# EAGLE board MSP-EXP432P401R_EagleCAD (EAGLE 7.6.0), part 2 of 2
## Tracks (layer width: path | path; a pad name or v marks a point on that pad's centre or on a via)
!RST  (via drill 0.3)
  Top 0.203: 54.61,34.29 v54.74,34.42 52.2,34.42 J2.16 | MSP1.83 26.72,23.74 26.29,23.3 25.08,23.3 24.57,22.8 24.57,19.37 24.89,19.05 39.75,19.05 40.96,20.26 45.53,20.26 46.1,19.68 56.2,19.68 57.53,21.02 v57.53,34.42 57.53,43.18 52.58,48.13 52.58,54.1 | J101.11 24.13,51.05 24.64,50.55 37.08,50.55 38.73,52.2 | 38.73,52.2 38.73,52.96 40.48,54.7 C13.1 R6.1 51.98,54.7 52.58,54.1 | 52.58,54.1 54.1,54.1 57.91,57.91 57.91,87.88 56.64,89.15 53.34,89.15 52.07,90.42 49.97,90.42 S3.S1 | J8.10 38.73,52.2
  Bottom 0.203: v57.53,34.42 v54.74,34.42
+3V3  (via drill 0.3)
  Top 0.203: MSP1.13 42.53,32.38 C4.1 42.94,32.77 v44.2,32.77 | v17.53,29.72 17.73,29.51 17.73,28.69 C7.1 17.73,26.73 C3.+ 18.6,27.38 MSP1.73 | R1.1 v19.05,43.31 | R6.2 51.31,53.38 v51.31,52.58
  Top 0.305: 18.91,26.81 C3.+
  Mid-Top 0.508: J5.35 J5.36 49.53,8.41 52.07,10.95 J6.1
  pour Mid-Top (isolate 0.254): 58.42,55.88 15.49,55.88 15.49,52.99 14.7,52.2 12.45,52.2 11.81,51.56 11.81,48.7 11.24,48.13 4.95,48.13 4.32,47.5 4.32,38.94 4.78,38.48 7.67,38.48 8.13,38.02 8.13,28.66 8.85,27.94 18.59,27.94 19.05,28.4 19.05,29.91 19.02,30.48 19.02,40.63 20.3,41.91 29.96,41.91 33.9,45.85 40.42,45.85 41.91,44.36 41.91,32.21 42.37,31.75 50.34,31.75 50.8,31.29 50.8,10.16 51.43,9.53 58.42,9.53
+5V  (via drill 0.3)
  Top 0.508: J5.33 J5.34 46.99,4.32 45.72,5.59 12.19,5.59 J7.1
  other vias: 8.13,49.91 9.4,49.91
  pour Mid-Top (isolate 0.61, rank 2): 0,55.88 14.99,55.88 14.99,53.57 14.37,52.96 11.79,52.96 11.05,52.22 11.05,49.81 10.51,49.28 4.3,49.28 3.56,48.54 3.56,38.35 4.19,37.72 6.83,37.72 7.37,37.19 7.62,9.99 7.16,9.53 0,9.53
  pour Bottom (isolate 0.254): 7.24,43.05 10.74,43.05 11.3,43.62 11.3,50.11 10.74,50.67 7.52,50.67 7.24,50.39
AVCC
  Top 0.203: MSP101.6 39.43,80.03 39.02,79.63 36.14,79.63 35.81,79.3 35.81,78.74 C116.2 35.77,78.71 35.72,78.71 R115.1 R114.2
AVCCOUT  (via drill 0.3)
  Top 0.203: R113.1 43.95,78.11 43.94,78.11 43.94,77.09 43.96,77.09 R112.2 | R113.1 44.16,78.99 v44.88,78.99 | 43.92,82.09 43.92,82.07 43.97,82.02 43.99,82.04 | 43.99,81.95 43.99,82.04 | 43.99,82.04 43.99,82.07 43.97,82.09 | C115.2 43.92,82.13 43.2,81.41 43.2,79.67 R113.1 | 43.81,78.97 43.9,78.97 R113.1 | MSP101.1 35.6,83.27 v35.56,83.57
  Top 0.508: C115.2 43.94,82.12 43.92,82.09
  Bottom 0.203: v35.56,83.57 35.56,82.3 37.34,80.52 43.36,80.52 v44.88,78.99
DCDCCAL0
  Top 0.203: R126.2 45.83,80.52 45.47,80.9 45.11,81.26 45.11,84.71 44.35,85.47 43.23,85.47 42.42,84.66 42.42,83.66 42.03,83.27 MSP101.12
DCDCCAL1  (via drill 0.3)
  Top 0.203: R127.2 45.8,77.64 45.8,78 45.8,78.46 45.82,78.49 45.8,78.49 v45.8,78.54 | MSP101.2 37.39,82.62 37.21,82.8 36.07,82.8 35.94,82.68 35.05,82.68 v34.92,82.55
  Bottom 0.203: v45.8,78.54 45.64,78.54 45.21,78.11 44.2,78.11 43.69,78.61 43.69,78.74 42.42,80.01 37.21,80.01 34.92,82.3 v34.92,82.55
DCDCCAL2
  Top 0.203: 41.62,82.63 MSP101.11 42.42,82.62 42.93,83.13 42.93,84.42 43.46,84.96 44.06,84.96 44.68,84.35 44.68,80.33 45.55,79.45 R128.2
DCDCIO0  (via drill 0.3)
  Top 0.203: MSP101.4 35.69,81.32 34.29,79.92 34.29,68.15 33.7,67.56 v30.73,67.56 | v21.46,68.2 20.83,68.83 12.66,68.83 11.81,67.98 IC106.P$5
  Bottom 0.203: v30.73,67.56 22.1,67.56 v21.46,68.2
DCDCIO1  (via drill 0.3)
  Top 0.203: MSP101.5 38.78,80.14 38.64,80.01 35.26,80.01 34.8,79.55 34.8,67.62 34.23,67.06 31.53,67.06 31.11,66.65 v30.86,66.55 | v20.07,68.2 12.83,68.2 12.21,67.58 IC106.P$6
  Bottom 0.203: v30.86,66.55 21.72,66.55 v20.07,68.2
DCDCPULSE  (via drill 0.3)
  Top 0.203: R118.2 45.82,84.95 v45.82,84.66 | MSP101.3 36.9,81.97 v36.83,82.04 35.59,82.04 33.78,80.24 33.78,69.25 32.86,68.33 30.35,68.33 v30.1,68.58 | v21.08,70.23 12.7,70.23 10.18,67.71 IC106.P$127
  Bottom 0.203: v36.83,82.04 37.72,81.15 42.32,81.15 v45.82,84.66 | v21.08,70.23 21.34,70.23 22.99,68.58 v30.1,68.58
DCDCRST  (via drill 0.3)
  Top 0.203: MSP101.9 41.91,81.32 42.19,81.04 42.19,78.64 TP108.1 42.16,77.85 38.48,74.17 36.2,74.17 v35.56,73.53 | IC106.P$11 14.21,64.91 14.73,64.39 18.41,64.39 v18.54,64.26
  Bottom 0.203: v18.54,64.26 18.8,64.26 19.94,65.41 35.56,65.41 36.07,65.91 36.07,67.56 35.56,68.07 v35.56,73.53
DCDCTEST  (via drill 0.3)
  Top 0.203: 41.73,81.97 41.66,82.04 41.66,81.92 MSP101.10 42.18,81.97 42.7,81.45 42.7,79.6 43.31,78.99 43.31,77.85 42.16,76.71 TP109.1 | TP109.1 | IC106.P$27 20.61,64.68 v20.07,64.14 | TP109.1 41.27,76.07 38.48,73.28 v36.7,73.28
  Bottom 0.203: v20.07,64.14 20.96,65.02 36.32,65.02 36.7,65.41 v36.7,73.28
DCOR
  Top 0.203: MSP1.44 26.21,41.1 24.13,43.18 R5.1
HOSTSCL  (via drill 0.3)
  Top 0.203: R117.2 39.15,78.65 39.88,79.38 v40,79.38 40.08,79.45 MSP101.7 | IC106.P$49 25,73.71 25.4,73.31 25.4,70.99 25.91,70.48 32.64,70.48 33.02,70.87 33.02,72.64 v32.77,72.9
  Bottom 0.203: v40,79.38 39.88,79.25 36.83,79.25 35.05,77.47 35.05,75.69 33.78,74.42 33.78,73.66 33.02,72.9 v32.77,72.9
HOSTSDA  (via drill 0.3)
  Top 0.203: 40.2,78.26 R116.2 40.28,78.26 v40.77,78.74 40.73,78.74 MSP101.8 | IC106.P$50 25.19,74.11 25.78,73.52 25.78,71.63 26.29,71.12 31.75,71.12 v32,71.37
  Bottom 0.203: v40.77,78.74 40.51,78.49 36.83,78.49 35.81,77.47 35.81,75.44 34.54,74.17 34.54,73.66 32.26,71.37 v32,71.37
IRSTN  (via drill 0.3)
  Top 0.203: R102.1 32.26,73.53 v30.48,71.76 | v4.7,72.77 3.43,72.77 TP106.1
  Bottom 0.203: v4.7,72.77 7.37,72.77 8.26,73.66 21.34,73.66 24.26,70.74 29.46,70.74 v30.48,71.76
ITCK
  Top 0.203: IC106.P$100 4.17,78.51 3.61,79.07 R129.1 2.84,79.72 2.54,80.01 2.54,80.77 1.27,82.04 TP103.1
ITDI  (via drill 0.3)
  Top 0.203: IC106.P$98 5.65,79.31 v5.33,79.63
  Bottom 0.203: v5.33,79.63 3.43,79.63 TP105.1
ITDO  (via drill 0.3)
  Top 0.203: IC106.P$97 6.27,79.71 v5.33,80.65
  Bottom 0.203: v5.33,80.65 1.9,80.65 TP104.1
ITMS
  Top 0.203: IC106.P$99 4.9,78.91 4.57,79.24 4.57,83.12 3.85,83.84 R125.1 2.38,85.09 TP102.1
LED0  (via drill 0.3)
  Top 0.203: IC106.P$3 11.01,64.61 v9.65,63.25 | R111.1 4.66,63.92 v4.83,63.75
  Bottom 0.203: v9.65,63.25 5.33,63.25 v4.83,63.75
LED1  (via drill 0.3)
  Top 0.203: IC106.P$4 11.41,64.5 10.54,63.63 v10.54,62.61 | v4.06,62.74 3.97,62.83 R124.1
  Bottom 0.203: v10.54,62.61 10.41,62.48 4.32,62.48 v4.06,62.74
N$1
  Top 0.254: JP102.2 48.39,59.56 J102.1
N$3
  Top 0.203: IC106.P$63 25.84,79.31 28.7,76.45 R108.2
N$4
  Top 0.203: R124.2 1.71,62.56 3.56,60.71 3.56,58.87 LED102.A
N$6  (via drill 0.3)
  Top 0.203: 32,22.29 C2.1 | 21.16,43.27 R1.2
  Top 0.305: 32,22.29 32,22.86 31.5,23.37 29.08,23.37 28.7,23.75 MSP1.87 28.7,26.12 28.47,26.35 v27.81,26.35 | 21.16,43.27 C1.1 22.73,42.67 23.37,42.04 24.64,42.04 25.71,40.97 MSP1.45 25.71,38.26 26.12,37.85 27.62,37.85 v27.81,38.04
  Bottom 0.305: v27.81,26.35 v27.81,38.04
N$7
  Top 0.203: LED101.A 2.72,60.53 2.29,60.96 1.27,60.96 0.76,61.47 0.76,63.5 1.18,63.92 R111.2
N$8
  Top 0.203: JP9.2 28.36,10.58 R2.1
N$9
  Top 0.203: R2.2 30.7,7.49 35.43,7.49 35.94,8 35.94,8.76 36.2,9.02 LED2.5
N$10
  Top 0.203: R3.2 32.86,7.87 35.18,7.87 35.56,8.26 35.56,9.27 36.03,9.74 LED2.6
N$11  (via drill 0.3)
  Top 0.203: R4.2 34.92,8.93 v34.92,9.65 | v36.58,7.49 36.66,7.58 LED2.4
  Bottom 0.203: v34.92,9.65 36.58,8 v36.58,7.49
N$12
  Top 0.305: R119.1 47.15,81.78 47.5,81.43 48.62,81.43 48.67,81.38 T102.E
N$13
  Top 0.305: T102.B 48.72,83.72 D101.2 D101.1 48.05,87.29 46.92,86.17 R118.1 46.8,85.74
N$15  (via drill 0.3)
  Top 0.635: D102.3 50.8,78.79 v51.61,79.38 | T101.3 55.37,81.05 v55.37,79.88 55.37,78.77 L101.1
  Bottom 0.635: v51.61,79.38 54.86,79.38 v55.37,79.88
N$16
  Top 0.203: 50.92,82.38 T102.C
  Top 0.305: T102.C 52.67,82.37 T101.1 | 50.98,82.32 50.92,82.38 D101.3 50.95,86.31 52.35,86.31 52.73,85.93 R120.2
N$17
  Top 0.203: LED1.A R7.2
N$19
  Top 0.203: JP10.2 30.9,10.58 R3.1
N$21
  Top 0.203: IC106.P$93 11.41,82.39 9.91,83.89 R138.2
N$22
  Top 0.203: IC106.P$61 24.99,78.51 26.92,76.58 R110.2
N$23
  Top 0.203: IC106.P$95 10.61,82.01 9.06,83.57 8.64,83.57 8.13,84.07 R131.2
N$24
  cutout Mid-Bottom: 11.68,86.28 17.53,86.36 17.53,82.27 11.66,82.25
  cutout Top: 11.68,86.28 17.53,86.36 17.53,82.27 11.66,82.25
  cutout Bottom: 11.68,86.28 17.53,86.36 17.53,82.27 11.66,82.25
  cutout Mid-Top: 11.68,86.28 17.53,86.36 17.53,82.27 11.66,82.25
N$25
  Top 0.203: JP11.2 33.44,10.58 R4.1
N$27
  Top 0.203: IC106.P$62 25.36,78.91 27.81,76.45 R109.2
N$29
  Top 0.254: JP8.2 24.13,9.17 R7.1
N$30
  cutout Top: 31.24,22.99 25.4,22.99 25.02,22.61 25.02,19.81 25.27,19.56 31.11,19.56 31.37,19.81 31.37,22.86
N$31
  cutout Mid-Top: 25.4,22.99 25.02,22.61 25.02,19.81 25.27,19.56 31.11,19.56 31.37,19.81 31.37,22.86 31.24,22.99
N$32
  cutout Mid-Bottom: 25.4,22.99 25.02,22.61 25.02,19.81 25.27,19.56 31.11,19.56 31.37,19.81 31.37,22.86 31.24,22.99
N$33
  cutout Bottom: 25.4,22.99 25.02,22.61 25.02,19.81 25.27,19.56 31.11,19.56 31.37,19.81 31.37,22.86 31.24,22.99
N$34
  Top 0.203: MSP1.42 27.2,41.38 26.49,42.09 Q1.1 26.47,43.46 C6.1
N$35
  cutout Mid-Top: 25.02,46.61 25.02,42.93 26.67,41.27 26.67,39.37 27.05,38.99 28.07,38.99 28.32,39.24 28.32,41.15 29.72,42.54 29.72,46.61 28.83,47.5 25.91,47.5
N$36
  cutout Mid-Bottom: 25.91,47.5 25.02,46.61 25.02,42.93 26.67,41.27 26.67,39.37 27.05,38.99 28.07,38.99 28.32,39.24 28.32,41.15 29.72,42.54 29.72,46.61 28.83,47.5
N$37
  cutout Bottom: 25.91,47.5 25.02,46.61 25.02,42.93 26.67,41.27 26.67,39.37 27.05,38.99 28.07,38.99 28.32,39.24 28.32,41.15 29.72,42.54 29.72,46.61 28.83,47.5
N$38
  Top 0.203: MSP1.41 27.71,41.43 28.4,42.11 Q1.2 28.35,43.48 C5.1
N$47
  Top 0.203: IC106.P$59 25.16,77.71 26.04,76.84 R139.2
OSC0
  Top 0.203: C102.1 16.58,85.6 Q101.3 15.24,85.6 14.61,84.96 14.61,83.19 13.41,81.99 IC106.P$88
OSC1
  Top 0.203: IC106.P$89 13.01,81.98 12.33,82.67 R106.2
OSC1_R
  Top 0.203: R106.1 13.51,83.17 Q101.1 12.58,84 C101.1
P1.0_LED1  (via drill 0.3)
  Top 0.203: v38.04,14.86 37.65,14.48 36.64,14.48 36.13,14.99 26.48,14.99 25.46,13.97 JP8.1 | MSP1.4 38.3,27.89 v38.35,27.94
  Bottom 0.203: v38.04,14.86 38.73,15.56 38.73,20.57 39.12,20.96 39.12,27.3 38.48,27.94 v38.35,27.94
P1.1_BUTTON1  (via drill 0.3)
  Top 0.203: MSP1.5 35.51,28.4 v35.05,27.94 | v17.53,42.67 17.53,45.21 9.91,52.83 S1.S1
  Mid-Top 0.203: v17.53,42.67 18.54,41.66 18.54,40.64 21.08,38.1 23.37,38.1 29.46,32 30.99,32 v35.05,27.94
P1.2_BCLUART_RXD  (via drill 0.3)
  Top 0.203: MSP1.6 35.21,28.88 34.42,29.68 34.42,36.07 34.92,36.58 v34.92,37.59 | v32.51,47.24 31.75,48.01 30.73,48.01 29.72,49.02 20.32,49.02 19.05,50.29 J101.7
  Mid-Top 0.203: v34.92,37.59 32.51,40 v32.51,47.24
P1.3_BCLUART_TXD  (via drill 0.3)
  Top 0.203: MSP1.7 35.76,29.39 34.8,30.35 34.8,35.5 v35.24,35.94 | v33.27,48.39 33.15,48.51 31.24,48.51 29.97,49.78 22.61,49.78 21.59,50.8 J101.9
  Mid-Top 0.203: v35.24,35.94 35.69,36.39 35.69,37.97 33.27,40.39 v33.27,48.39
P1.4_BUTTON2  (via drill 0.3)
  Top 0.203: MSP1.8 37.92,29.9 v38.61,29.21 | v42.67,43.18 46.48,46.99 v49.78,46.99 | S2.S1 55.12,48.2 v55.12,46.74
  Mid-Top 0.203: v38.61,29.21 38.61,30.99 42.16,34.54 42.16,42.67 v42.67,43.18
  Bottom 0.203: v49.78,46.99 50.04,46.74 v55.12,46.74
P1.5_SPICLK_J1.7  (via drill 0.3)
  Top 0.203: v40.13,12.51 38.42,12.51 38.04,12.89 20.7,12.89 20.19,12.38 11.43,12.38 9.08,14.73 9.08,18.61 8.38,19.3 5.02,19.3 4.38,19.94 4.38,28.26 5.33,29.21 J1.7 | MSP1.9 39.22,30.38 39.5,30.1 39.5,27.69 v40.89,26.29
  Bottom 0.203: v40.13,12.51 40.7,13.08 40.7,14.73 40.89,14.92 v40.89,26.29
P1.6_SPIMOSI_J2.15  (via drill 0.3)
  Top 0.203: v48.01,30.29 48.2,30.48 50.8,30.48 J2.15 | MSP1.10 39.22,30.89 39.88,30.23 39.88,27.81 40.64,27.05 47.43,27.05 v47.75,26.73
  Bottom 0.203: v47.75,26.73 48.01,26.99 v48.01,30.29
P1.7_SPIMISO_J2.14
  Top 0.203: MSP1.11 39.22,31.39 40.26,30.35 40.26,27.94 40.64,27.56 44.45,27.56 44.83,27.94 50.8,27.94 J2.14
P2.0_RGBLED_RED  (via drill 0.3)
  Top 0.203: v29.84,32.96 29.84,30.54 26.23,26.92 24.07,26.92 20.7,23.56 20.7,22.1 21.4,21.4 v21.59,21.4 | MSP1.16 37.68,33.88 37.99,33.58 v39.05,33.58
  Bottom 0.203: v39.05,33.58 38.48,32.96 v29.84,32.96 | v21.59,21.4 21.78,21.21 21.78,16.13 22.67,15.24 27.88,15.24 29.15,13.97 JP9.1
P2.1_RGBLED_GREEN  (via drill 0.3)
  Top 0.203: MSP1.17 38.19,34.39 v38.35,34.23 | v29.96,33.92 29.65,33.92 29.08,33.4 29.08,30.35 26.04,27.3 23.88,27.3 19.94,23.37 19.94,22.1 20.64,21.4 v20.64,21.15
  Bottom 0.203: v38.35,34.23 36.77,34.23 35.94,33.4 30.48,33.4 v29.96,33.92 | v20.64,21.15 21.27,20.51 21.27,14.92 23.3,12.89 30.29,12.89 31.37,13.97 JP10.1
P2.2_RGBLED_BLUE  (via drill 0.3)
  Top 0.203: v39.37,34.73 39.26,34.87 39.14,34.99 37.85,34.99 37.72,34.86 37.34,34.86 37.32,34.87 MSP1.18 | v29.84,35.05 28.45,33.65 28.45,30.42 26.61,28.57 v23.81,28.57 | v20.7,25.46 20.45,25.46 19.56,24.57 v19.56,20.96
  Bottom 0.203: v29.84,35.05 30.16,35.05 31.37,33.84 35.69,33.84 36.83,34.99 39.18,34.99 v39.37,34.73 | v19.56,20.96 20.83,19.68 20.83,14.48 22.8,12.51 33.15,12.51 34.29,13.65 JP11.1 | v23.81,28.57 v20.7,25.46
P2.3_IO_J4.34
  Top 0.203: MSP1.19 39.8,35.38 40.51,34.67 42.25,34.67 43.08,33.84 44.64,33.84 45.02,33.46 45.02,30.54 46.35,29.21 J4.34
P2.4_PWM_J4.38
  Top 0.203: MSP1.20 39.19,35.89 42.67,39.37 J4.38
P2.5_PWM_J2.19
  Top 0.203: MSP1.21 39.04,36.37 43.31,40.64 50.8,40.64 J2.19
P2.6_PWM_J4.39
  Top 0.203: MSP1.22 38.91,36.88 43.94,41.91 J4.39
P2.7_PWM_J4.40
  Top 0.203: MSP1.23 38.72,37.39 45.78,44.45 J4.40
P3.0_IO_J2.18  (via drill 0.3)
  Top 0.203: MSP1.32 32.21,41.86 34.29,43.94 37.59,43.94 40.51,41.02 v41.02,41.02
  Bottom 0.203: v41.02,41.02 44.58,41.02 47.5,38.1 50.8,38.1 J2.18
P3.2_URXD_J1.3  (via drill 0.3)
  Top 0.203: MSP1.34 31.22,38.01 29.65,36.45 v26.92,36.45 | v13.46,38.54 11.37,40.64 7.62,40.64 J1.3 | v21.46,39.12 17.34,39.12 v17.08,38.86
  Bottom 0.203: v17.08,38.86 13.78,38.86 v13.46,38.54 | v26.92,36.45 24.13,36.45 v21.46,39.12
P3.3_UTXD_J1.4  (via drill 0.3)
  Top 0.203: MSP1.35 30.71,38.2 29.59,37.08 v26.16,37.08 | v16.19,38.23 16.19,39.24 17.08,40.13 v22.1,40.13 | v11.56,37.85 11.3,38.1 7.62,38.1 J1.4
  Bottom 0.203: v11.56,37.85 15.81,37.85 v16.19,38.23 | v26.16,37.08 25.15,37.08 v22.1,40.13
P3.5_IO_J4.32
  Top 0.203: MSP1.37 29.72,40.96 36.77,48.01 50.6,48.01 55.63,42.98 55.63,23.37 55.12,22.86 50.8,22.86 J4.32
P3.6_IO_J2.11
  Top 0.203: MSP1.38 29.21,40.96 36.7,48.45 50.87,48.45 56.2,43.12 56.2,22.16 55.63,21.59 J2.11
P3.7_IO_J4.31
  Top 0.203: MSP1.39 28.77,41.02 36.7,48.96 51.04,48.96 56.77,43.23 56.77,21.34 55.75,20.32 50.8,20.32 J4.31
P4.0_A13_J3.24
  Top 0.203: MSP1.56 11.67,35.89 10.73,36.83 J3.24
P4.1_IO_J1.5
  Top 0.203: MSP1.57 10.91,35.38 10.73,35.56 7.62,35.56 J1.5
P4.2_A11_J3.25
  Top 0.203: MSP1.58 9.47,34.87 J3.25
P4.3_A10_J1.6
  Top 0.203: MSP1.59 12.68,34.39 11.3,33.02 7.62,33.02 J1.6
P4.4_A9_J3.26
  Top 0.203: MSP1.60 13.12,33.88 10.92,31.69 8.95,31.69 J3.26
P4.5_A8_J3.27
  Top 0.203: MSP1.61 14.9,33.38 10.73,29.21 J3.27
P4.6_IO_J1.8
  Top 0.203: MSP1.62 15.37,32.89 10.41,27.94 7.62,27.94 J1.8
P4.7_A6_J3.28
  Top 0.203: MSP1.63 15.81,32.38 10.1,26.67 J3.28
P5.0_IO_J2.13  (via drill 0.3)
  Top 0.203: MSP1.64 24.89,31.88 26.92,29.84 v26.92,29.78 | v24.77,17.14 46.35,17.14 46.99,17.78 v46.99,18.35 | v47.05,25.34 50.74,25.34 J2.13
  Bottom 0.203: v46.99,18.35 46.99,25.15 v47.05,25.34 | v24.77,17.14 23.62,17.14 23.11,17.65 23.11,22.48 24,23.37 24,26.35 24.77,27.11 25.02,27.11 26.92,29.02 v26.92,29.78
P5.1_IO_J4.33  (via drill 0.3)
  Top 0.203: v23.88,16.51 46.48,16.51 47.62,17.65 v47.62,19.05 | MSP1.65 24.49,31.39 26.04,29.84 v26.04,29.21
  Bottom 0.203: v47.62,19.05 47.62,24.77 J4.33 | v23.88,16.51 23.5,16.51 22.73,17.27 22.73,22.61 23.62,23.5 23.62,26.54 26.04,28.96 v26.04,29.21
P5.2/XT2IN
  Top 0.203: MSP1.86 28.22,23.47 29.29,22.39 Q2.1 | 29.21,22.35 Q2.1 | C12.1 29.48,22.32 Q2.1
P5.2_IO_J2.12  (via drill 0.3)
  Top 0.203: MSP1.66 23.85,30.89 v25.08,29.65 | v25.08,15.88 46.48,15.88 48.32,17.72 v48.32,18.29
  Bottom 0.203: v48.32,18.29 48.32,22.36 48.82,22.86 50.8,22.86 J2.12 | v25.08,15.88 23.37,15.88 22.29,16.95 22.29,22.8 23.24,23.75 23.24,26.8 25.08,28.64 v25.08,29.65
P5.3  (via drill 0.3)
  Top 0.203: MSP1.67 20.68,30.38 v19.68,31.37
  Bottom 0.203: v19.68,31.37 14.86,31.37 14.1,30.61 14.1,18.54 11.05,15.49 11.05,8.89 15.24,4.7 15.24,2.54 J5.9
P5.3/XT2OUT
  Top 0.203: MSP1.85 27.71,23.34 28.19,22.86 28.19,21.33 27.4,20.54 Q2.3 26.91,20.36 C11.1
P5.4_IO_J3.29
  Top 0.203: MSP1.68 20.08,29.9 18.73,31.24 16,31.24 12.38,27.62 12.38,25.08 11.43,24.13 J3.29
P5.5_IO_J3.30
  Top 0.203: MSP1.69 19.89,29.39 18.54,30.73 16.45,30.73 13.27,27.56 13.27,22.92 11.94,21.59 J3.30
P5.6_PWM_J4.37  (via drill 0.3)
  Top 0.203: v40.32,36.07 41.08,36.83 J4.37 | MSP1.70 22.53,28.88 22.86,29.21 22.86,29.91 v23.18,30.23 | v25.72,32.77 25.97,32.77 29.21,36.07 30.58,36.07 v31.22,35.43
  Bottom 0.203: v40.32,36.07 36.39,36.07 35.5,35.18 32.77,35.18 32.51,35.43 v31.22,35.43 | v25.72,32.77 v23.18,30.23
P5.7_IO_J2.17  (via drill 0.3)
  Top 0.203: v41.02,35.37 41.27,35.56 50.8,35.56 J2.17 | v32.13,34.61 30.8,34.61 30.54,34.86 30.54,35.43 30.29,35.69 29.53,35.69 25.96,32.12 v25.96,31.8 | MSP1.71 22.68,28.4 23.81,29.53 v24,29.53
  Bottom 0.203: v32.13,34.61 35.62,34.61 36.39,35.37 v41.02,35.37 | 25.96,31.67 v25.96,31.8 25.96,31.48 v24,29.53
P6.0_A15_J1.2
  Top 0.203: MSP1.54 16.65,36.88 10.35,43.18 7.56,43.18 6.35,41.97 J1.2
P6.1_A14_J3.23
  Top 0.203: MSP1.55 14.24,36.37 11.24,39.37 J3.23
P6.2  (via drill 0.3)
  Top 0.203: MSP1.76 23.22,24.61 v21.97,23.37
  Bottom 0.203: v21.97,23.37 16.38,23.37 15.49,22.48 15.49,18.03 12.45,14.99 12.45,9.65 16.26,5.84 17.27,5.84 19.05,4.06 J5.12
P6.3  (via drill 0.3)
  Top 0.203: MSP1.77 23.7,23.82 22.35,22.48 v21.34,22.48
  Bottom 0.203: v21.34,22.48 16.51,22.48 16,21.97 16,17.78 12.83,14.61 12.83,9.91 16.38,6.35 18.41,6.35 20.32,4.45 20.32,2.41 21.46,1.27 J5.13
P6.4_I2CSDA_J1.10
  Top 0.203: MSP1.78 24.21,23.64 23.75,23.18 23.75,21.34 22.73,20.32 7.62,20.32 J1.10
P6.5_I2CSCL_J1.9
  Top 0.203: MSP1.79 24.71,23.44 24.13,22.86 24.13,21.08 22.86,19.81 5.84,19.81 5.08,20.57 5.08,22.86 J1.9
P6.6_CAPTURE_J4.36  (via drill 0.3)
  Top 0.203: v23.94,17.78 45.47,17.78 46.16,18.48 v46.16,18.99 | v47.05,32.51 47.05,33.84 47.5,34.29 J4.36 | MSP1.80 25.22,25.58 v24.83,26.16
  Bottom 0.203: v24.83,26.16 24.83,23.62 23.5,22.29 23.5,18.22 v23.94,17.78 | v47.05,32.51 47.24,32.32 47.24,27.18 46.42,26.35 46.42,19.24 v46.16,18.99
P6.7_CAPTURE_J4.35  (via drill 0.3)
  Top 0.203: MSP1.81 25.71,26.21 v25.78,26.29 | v46.55,30.99 47.31,31.75 J4.35 | v45.27,19.43 44.26,18.41 v24.64,18.41
  Bottom 0.203: v25.78,26.29 25.78,24.07 24.07,22.35 24.07,18.99 v24.64,18.41 | v46.55,30.99 46.74,30.8 46.74,27.3 45.78,26.35 45.78,19.88 45.34,19.43 v45.27,19.43
P7.0  (via drill 0.3)
  Top 0.203: MSP1.88 29.21,26.54 v28.7,27.05
  Mid-Top 0.203: v28.7,27.05 24.77,27.05 17.65,19.94 17.65,8.64 19.94,6.35 23.37,6.35 25.4,4.32 25.4,2.67 26.67,1.4 J5.17
P7.1  (via drill 0.3)
  Top 0.203: MSP1.89 29.72,27.18 v28.7,28.19
  Mid-Top 0.203: v28.7,28.19 28.45,28.19 27.69,27.43 24.64,27.43 17.27,20.07 17.27,8.38 19.68,5.97 22.1,5.97 24.13,3.94 J5.16
P7.2  (via drill 0.3)
  Top 0.203: MSP1.90 30.2,27.58 v29.84,27.94
  Mid-Top 0.203: v29.84,27.94 29.84,28.32 29.34,28.83 28.32,28.83 27.3,27.81 24.51,27.81 16.89,20.19 16.89,8.13 19.43,5.59 21.46,5.59 22.86,4.19 22.86,2.41 24,1.27 J5.15
P7.3  (via drill 0.3)
  Top 0.203: MSP1.91 30.71,28.47 v29.84,29.34
  Mid-Top 0.203: v29.84,29.34 28.32,29.34 27.18,28.19 24.38,28.19 16.51,20.32 16.51,7.87 19.3,5.08 20.45,5.08 21.59,3.94 J5.14
P7.4  (via drill 0.3)
  Top 0.203: MSP1.26 35.71,40.51 v36.07,40.51
  Mid-Top 0.203: J5.24 34.29,4.57 36.58,6.86 40.26,6.86 41.66,8.26 41.66,19.81 36.2,25.27 36.2,35.31 36.96,36.07 36.96,39.62 v36.07,40.51
P7.5  (via drill 0.3)
  Top 0.203: MSP1.27 34.72,40.95 35.05,41.27 v36.96,41.27
  Mid-Top 0.203: J5.23 35.56,2.54 35.56,4.57 37.46,6.48 40.51,6.48 42.04,8 42.04,20.07 36.58,25.53 36.58,35.18 37.34,35.94 37.34,40.77 36.96,41.15 v36.96,41.27
P7.6  (via drill 0.3)
  Top 0.203: MSP1.28 34.21,41.58 34.54,41.91 v36.07,41.91
  Mid-Top 0.203: J5.26 36.83,4.57 38.35,6.1 40.77,6.1 42.42,7.75 42.42,20.32 36.96,25.78 36.96,35.05 37.72,35.81 37.72,39.88 38.23,40.39 38.23,41.53 37.85,41.91 v36.07,41.91
P7.7  (via drill 0.3)
  Top 0.203: MSP1.29 33.71,42.09 34.16,42.54 36.83,42.54 v36.96,42.67
  Mid-Top 0.203: J5.25 38.1,2.54 38.1,4.57 39.24,5.71 41.02,5.71 42.8,7.49 42.8,20.57 37.34,26.04 37.34,34.92 38.1,35.69 38.1,39.75 38.61,40.26 38.61,42.16 38.1,42.67 v36.96,42.67
P8.0  (via drill 0.3)
  Top 0.203: MSP1.30 33.2,42.34 34.29,43.43 35.81,43.43 v36.07,43.18
  Mid-Top 0.203: v36.07,43.18 36.45,43.56 38.23,43.56 38.99,42.8 38.99,40 38.48,39.5 38.48,35.43 37.72,34.67 37.72,26.29 43.18,20.83 43.18,12.83 v43.69,12.32
  Bottom 0.203: v43.69,12.32 43.69,12.07 40,8.38 39.5,8.38 36.32,5.21 33.27,5.21 31.88,3.81 J5.22
P8.2  (via drill 0.3)
  Top 0.203: MSP1.46 25.22,35.64 v24.89,35.31
  Bottom 0.203: v24.89,35.31 24.89,35.05 24.13,34.29 14.35,34.29 13.59,33.53 13.59,18.8 10.54,15.75 10.54,7.37 13.97,3.94 J5.8
P8.3  (via drill 0.3)
  Top 0.203: MSP1.47 24.71,36.27 v23.5,35.05
  Bottom 0.203: v23.5,35.05 13.46,35.05 13.08,34.67 13.08,19.05 10.03,16 10.03,6.99 12.7,4.32 12.7,2.41 13.84,1.27 J5.7
P8.4  (via drill 0.3)
  Top 0.203: MSP1.48 24.21,36.91 v23.37,36.07
  Bottom 0.203: v23.37,36.07 13.34,36.07 12.57,35.31 12.57,19.3 9.53,16.26 9.53,6.22 11.43,4.32 J5.6
P8.5  (via drill 0.3)
  Top 0.203: MSP1.49 23.7,40.95 22.99,41.66 13.84,41.66 v13.72,41.53
  Bottom 0.203: v13.72,41.53 11.43,41.53 10.16,40.26 10.16,20.19 7.62,17.65 7.62,10.54 6.22,9.14 6.22,3.94 J5.2
P8.6  (via drill 0.3)
  Top 0.203: MSP1.50 23.22,40.66 22.73,41.15 14.86,41.15 v14.22,40.51
  Bottom 0.203: v14.22,40.51 11.94,40.51 10.67,39.24 10.67,19.94 8,17.27 8,10.29 7.37,9.65 7.37,2.29 J5.1
P8.7  (via drill 0.3)
  Top 0.203: MSP1.51 20.8,38.38 20.45,38.73 18.41,38.73 v18.16,38.48
  Bottom 0.203: v18.16,38.48 17.78,38.48 16.64,37.34 12.19,37.34 11.18,36.32 11.18,19.81 8.38,17.02 8.38,9.91 7.75,9.27 7.75,2.54 8.89,1.4 J5.3
P9.0  (via drill 0.3)
  Top 0.203: v18.54,37.59 19.18,38.23 20.19,38.23 20.52,37.9 MSP1.52
  Bottom 0.203: v18.54,37.59 17.65,37.59 16.89,36.83 12.32,36.83 11.68,36.2 11.68,19.68 8.76,16.76 8.76,3.94 J5.4
P9.1  (via drill 0.3)
  Top 0.203: MSP1.53 20.02,37.39 v19.81,37.59
  Bottom 0.203: v19.81,37.59 19.68,37.59 18.54,36.45 12.57,36.45 12.19,36.07 12.19,19.56 9.14,16.51 9.14,5.97 10.16,4.95 10.16,2.41 11.3,1.27 J5.5
P9.2  (via drill 0.3)
  Top 0.203: MSP1.74 20.52,26.87 19.18,25.53 v17.91,25.53
  Bottom 0.203: v17.91,25.53 16.38,25.53 14.61,23.75 14.61,18.41 11.56,15.37 11.56,9.14 16.51,4.19 J5.10
P9.3  (via drill 0.3)
  Top 0.203: MSP1.75 20.68,26.39 18.92,24.64 v18.8,24.64
  Bottom 0.203: v18.8,24.64 16.13,24.64 14.99,23.5 14.99,18.16 11.94,15.11 11.94,9.53 16.13,5.33 16.76,5.33 17.78,4.32 17.78,2.54 J5.11
P9.4  (via drill 0.3)
  Top 0.203: MSP1.96 33.2,23.55 v32.89,23.24
  Mid-Top 0.203: v32.89,23.24 32.89,19.68 32,18.8 27.3,18.8 25.78,17.27 25.78,4.95 26.67,4.06 J5.18
P9.5  (via drill 0.3)
  Top 0.203: MSP1.97 33.71,22.53 v33.65,22.48
  Mid-Top 0.203: v33.65,22.48 33.65,19.81 32.13,18.29 27.56,18.29 26.29,17.02 26.29,5.97 27.94,4.32 27.94,2.41 29.08,1.27 J5.19
P9.6  (via drill 0.3)
  Top 0.203: MSP1.98 34.21,22.94 v34.8,22.35
  Mid-Top 0.203: v34.8,22.35 34.8,20.32 32.26,17.78 27.81,17.78 26.8,16.76 26.8,6.35 29.21,3.94 J5.20
P9.7  (via drill 0.3)
  Top 0.203: MSP1.99 34.72,23.44 v35.94,22.23
  Mid-Top 0.203: v35.94,22.23 35.94,20.83 32.38,17.27 28.07,17.27 27.3,16.51 27.3,6.6 28.83,5.08 29.84,5.08 30.48,4.45 30.48,2.29 31.5,1.27 J5.21
P10.0  (via drill 0.3)
  Top 0.203: MSP1.100 35.2,23.98 v35.81,23.37
  Mid-Top 0.203: v35.81,23.37 36.58,22.61 38.23,22.61 41.27,19.56 41.27,9.27 v39.62,7.62
  Bottom 0.203: v39.62,7.62 39.62,4.06 J5.28
P10.1  (via drill 0.3)
  Top 0.203: MSP1.1 37.62,26.39 38.35,25.65 38.35,24.64 39.75,23.24 v41.78,23.24
  Bottom 0.203: v41.78,23.24 42.54,22.48 42.54,18.54 45.59,15.49 45.59,13.21 40.64,8.26 40.64,2.54 J5.27
P10.2  (via drill 0.3)
  Top 0.203: MSP1.2 37.77,26.87 38.86,25.78 38.86,25.02 39.75,24.13 v42.54,24.13
  Bottom 0.203: v42.54,24.13 43.05,23.62 43.05,18.67 46.1,15.62 46.1,12.83 41.91,8.64 J5.30
P10.3  (via drill 0.3)
  Top 0.203: MSP1.3 37.9,27.38 39.37,25.91 39.37,25.4 39.88,24.89 v43.31,24.89
  Bottom 0.203: v43.31,24.89 43.56,24.64 43.56,18.8 46.61,15.75 46.61,12.45 43.18,9.02 43.18,2.54 J5.29
P10.4  (via drill 0.3)
  Top 0.203: MSP1.24 37.9,37.9 v39.12,39.12
  Bottom 0.203: v39.12,39.12 44.58,39.12 45.34,38.35 45.34,27.3 44.07,26.04 44.07,18.92 47.12,15.88 47.12,12.19 44.45,9.53 J5.32
P10.5  (via drill 0.3)
  Top 0.203: MSP1.25 37.11,38.38 38.61,39.88 40,39.88 v40.13,40
  Bottom 0.203: v40.13,40 44.7,40 45.85,38.86 45.85,27.18 44.58,25.91 44.58,19.05 47.62,16 47.62,11.81 45.72,9.91 45.72,2.54 J5.31
P96VBUS
  Top 0.254: IC106.P$96 10.21,81.74 9.14,82.8 7.68,82.8 C150.1 7.56,82.8 R140.2
REF_MAIN_LDO
  Top 0.203: IC106.P$128 7.62,67.31 7.21,66.9 R135.2 R136.2
REF_TARGET_VCC  (via drill 0.3)
  Top 0.203: R101.2 R134.2 42.42,71.88 36.2,65.66 34.16,65.66 v33.53,66.29 | v21.08,71.37 12.45,71.37 v11.94,70.87 | v10.16,70.61 10.06,70.51 IC106.P$120
  Bottom 0.203: v21.08,71.37 22.48,69.98 30.73,69.98 33.53,67.18 v33.53,66.29 | v11.94,70.87 10.41,70.87 v10.16,70.61
TCK_SWDCLK  (via drill 0.3)
  Top 0.203: MSP1.95 32.7,24.78 32.7,26.86 34.04,28.19 34.04,36.64 v33.97,36.7 | v37.85,47.24 41.91,47.24 v42.67,46.48
  Bottom 0.203: v33.97,36.7 33.97,43.75 35.05,44.83 40.26,44.83 42.04,46.61 | 42.04,46.61 44.45,49.02 J8.4 | J101.15 30.73,53.09 32.26,53.09 34.29,51.05 34.29,49.15 36.2,47.24 v37.85,47.24 | v42.67,46.48 42.54,46.61 42.04,46.61
TDI  (via drill 0.3)
  Top 0.203: MSP1.92 31.22,27.41 32.89,29.08 32.89,34.8 v31.05,36.64 | v31.75,45.21 v35.94,49.4 41.27,49.4 41.91,50.04 J8.8 | v35.94,51.43 34.29,53.09 J101.19
  Bottom 0.203: v31.75,45.21 31.75,42.42 31.11,41.78 31.11,36.7 v31.05,36.64 | v35.94,49.4 v35.94,51.43
TDO_SWO  (via drill 0.3)
  Top 0.203: MSP1.93 31.75,24.82 31.75,27.11 33.27,28.64 33.27,35.43 v32.58,36.13
  Bottom 0.203: v32.58,36.13 32,36.7 32,39.24 32.89,40.13 32.89,44.2 34.54,45.85 37.72,45.85 40,48.13 | J101.17 31.75,54.36 35.05,51.05 35.05,49.02 35.94,48.13 40,48.13 | 40,48.13 43.18,51.31 J8.6
TMS_SWDIO  (via drill 0.3)
  Top 0.203: MSP1.94 32.2,24.78 32.2,26.92 33.65,28.38 33.65,36.07 33.02,36.7 v33.02,37.1 | v43.43,49.78 45.72,52.07 J8.2 | v36.83,46.48 v39.62,46.48
  Bottom 0.203: v33.02,37.1 33.02,39.37 33.53,39.88 33.53,44.07 34.8,45.34 39.56,45.34 40.16,45.94 | v43.43,49.78 43.43,49.21 40.16,45.94 | J101.13 32,49.28 33.53,49.28 36.32,46.48 v36.83,46.48 | v39.62,46.48 40.16,45.94
VBUS_DETECT
  Top 0.203: IC106.P$1 10.21,64.82 8.76,63.37 8.76,62.09 R132.2 R133.2
VCCEN1  (via drill 0.3)
  Top 0.203: R107.1 45.52,75.61 45.21,75.3 v45.21,74.55 44.2,73.53 TP110.1 v34.92,66.29 | IC106.P$78 17.41,80.25 v17.91,79.76 | v17.91,78.11 17.91,75.69 v21.21,72.39 | IC103.1 54.47,73.6 v55.17,72.9
  Bottom 0.203: v45.21,74.55 46.23,73.53 54.53,73.53 v55.17,72.9 | v17.91,79.76 v17.91,78.11 | v21.21,72.39 23.24,70.36 31.11,70.36 34.92,66.55 v34.92,66.29
VCORE
  Top 0.305: MSP1.12 40.84,31.88 L1.1 41.27,30.21 C8.1 41.18,28.93
  Top 0.406: 41.18,28.93 C10.1
VDDC  (via drill 0.3)
  Top 0.203: 6.34,70.46 C132.2 | v10.16,72.39 10.16,72.51 IC106.P$115 7.23,72.51 C131.1 6.67,71.46 C132.2 | IC106.P$87 13.81,77.38 v13.84,77.34 | v13.97,75.44 13.97,75.06 v11.81,72.9 | C133.1 6.67,68.96 C132.2
  Bottom 0.203: v10.16,72.39 11.3,72.39 v11.81,72.9 | v13.84,77.34 13.84,75.56 v13.97,75.44
VREFA+
  Top 0.203: IC106.P$9 13.41,64.69 13.84,64.26 14.22,64.26 14.86,63.63 15.33,63.63 R105.1 C111.1 C110.1 19.01,63.54 20.17,62.38 IC107.3
VSW
  Top 0.305: MSP1.14 40.84,32.89 L1.2
XDS-GND  (via drill 0.3)
  Top 0.203: MSP1.40 28.22,38.92 28.34,38.8 28.87,38.8 29.08,38.58 v29.64,38.58 | MSP1.43 v26.72,38.52 | C11.2 v25.65,22.48 | C12.2 v30.73,20.19 | MSP1.84 27.2,25.91 v26.78,26.33 | MSP1.15 35.48,33.38 v35.48,32.11 | MSP1.72 20.14,27.89 v19.55,28.49 | v53.45,54.84 57.4,58.79 57.4,87.63 56.39,88.65 53.09,88.65 52.07,89.66 49.11,89.66 v48.63,90.15
  Top 0.254: MSP1.82 26.21,25.76 v26.78,26.33
  Top 0.406: C6.2 26.88,46.99 v27.43,46.99 27.91,46.99 C5.2 | 41.77,93.47 v41.77,93.45 | S3.S2 44.44,91.63 | 51.55,93.47 v51.55,93.45 | v48.63,90.15 v44.44,90.15 | S3.G2 42.93,93.47
  Top 0.635: S3.G2 41.77,93.47 | 44.44,91.63 v44.44,90.15 | S3.G1 51.55,93.47
  Mid-Bottom 0.203: v25.65,22.48 25.65,23.24 26.78,24.37 v26.78,26.33 | v30.73,20.19 30.86,20.07 v32,20.07 | v27.43,48.13 v27.43,46.99
  Bottom 0.406: v44.44,90.15 44.35,90.15 41.77,92.72 v41.77,93.45 | v48.63,90.15 51.55,93.07 v51.55,93.45
  other vias: 22.73,45.59 15.42,28.55 15.34,25.79 19.1,9.12 39.1,8.93 43.48,30.07 4.69,51.03 53.71,50.77 49.96,52.43 57.39,45.95 3.16,54.84 2.91,46.08
  pour Mid-Bottom (isolate 0.254): 0,55.63 58.42,55.63 58.42,0 0,0
  pour Top (isolate 0.254): 58.42,55.63 58.42,0 0,0 0,55.63
  cutout Top: 25.91,47.5 25.02,46.61 25.02,42.93 26.67,41.27 26.67,39.37 27.05,38.99 28.07,38.99 28.32,39.24 28.32,41.15 29.72,42.54 29.72,46.61 28.83,47.5
XDSET_!RST  (via drill 0.3)
  Top 0.203: C108.1 R102.2 R103.2 31.37,76.84 v31.11,77.09 | IC106.P$70 20.61,80.17 v20.19,79.76
  Bottom 0.203: v20.19,79.76 21.08,79.76 22.73,78.11 30.1,78.11 v31.11,77.09
XDSET_DM  (via drill 0.3)
  Top 0.203: R138.1 9.91,85.85 8.89,86.87 v9.02,87.12 | IC102.5 11.32,88 10.92,88.39 v10.79,88.39 10.78,88.41 USB101.D-
  Bottom 0.203: v9.02,87.12 9.53,87.12 v10.79,88.39
XDSET_DP  (via drill 0.3)
  Top 0.203: USB101.D+ 11.43,88.9 v11.94,88.39 11.94,87.61 IC102.4 | R137.1 9.02,85.73 v7.87,86.87
  Bottom 0.203: v7.87,86.87 8.26,86.49 10.03,86.49 v11.94,88.39
XDSET_DPR
  Top 0.203: IC106.P$94 11.01,82.2 9.02,84.19 R137.2
XDSET_GND  (via drill 0.3, 0.51)
  Top 0.203: IC102.3 13.2,86.74 v13.34,86.87 | LED101.C 0.81,59.53 v0.81,59 0.81,58.43 LED102.C | C101.2 12.19,85.26 v12.19,85.85 | C102.2 17.02,84.28 v17.02,83.19 | IC101.4 25.54,87.58 IC101.9 | MSP101.TP 40.08,82.62 MSP101.14
  Top 0.406: USB101.GND 12.73,89.25 13.46,88.52 v13.72,88.52 v14.73,88.52
  Mid-Bottom 0.203: v12.19,85.85 12.19,85.73 11.94,85.73 v11.05,84.84 | v17.02,83.19 v18.16,83.19
  other vias: 43.69,86.74 45.97,87.12 50.04,85.22 16.76,61.72 13.72,61.72 49.91,79.5 19.05,82.68 11.43,60.96 29.34,73.79 55.75,82.68 51.82,84.96 50.8,81.28 50.04,83.44 47.62,78.49 17.65,60.45 8.38,66.17 49.78,66.55 4.7,77.72 6.22,89.66 39.12,82.8 43.81,84.2 11.43,76.2 30.99,80.52 45.97,83.31 40.39,81.79 55.37,87.12 51.18,77.09 53.85,72.77 55.37,75.95 54.99,67.82 26.92,74.17 50.67,69.85 8.13,59.56 40.13,67.06 43.94,81.03 38.1,71.88 31.5,63.5 33.27,88.9 47.37,72.77 47.37,71.76 47.24,57.91 55.12,60.45 24.26,84.2 21.59,84.84 7.62,81.15 23.75,89.92 26.04,88.77 28.57,89.92 25.4,80.39 22.61,76.07 22.73,73.66 5.21,74.17 3.94,69.6 4.45,71.63 6.1,61.85 16.26,79.63 13.97,67.18 17.27,67.44 22.1,61.72 32.89,74.04 37.85,77.72 18.92,92.2 38.23,92.96
  pour Top: 0,95.25 58.42,95.25 58.42,56.64 0,56.64
  pour Mid-Bottom: 0,95.25 58.42,95.25 58.42,56.64 0,56.64
XDSET_ID  (via drill 0.3)
  Top 0.203: USB101.ID 12.08,89.14 12.7,88.52 v12.7,87.63 | v7.49,85.98 8.13,85.6 R131.1 | IC102.2 11.32,86.23 11.3,86.23 v10.92,85.85
  Bottom 0.203: v12.7,87.63 v10.92,85.85 10.79,85.98 v7.49,85.98
XDSET_RESET_OUT
  Top 0.203: IC106.P$40 28.31,70.11 28.96,69.47 28.96,62.48 29.21,62.23 | 29.21,62.23 36.58,62.23 39.62,59.18 39.62,58.67 40,58.29 J102.10 | 29.21,62.23 J101.12
XDSET_RXD
  Top 0.203: IC106.P$33 25.14,67.31 25.4,67.06 25.4,64.01 24.64,63.25 24.64,60.2 J101.10
XDSET_SHIELD  (via drill 0.3)
  Top 0.203: IC102.1 10.52,86.76 9.53,87.76 v8.26,87.76 | USB101.SHIELD_TH2 16.56,91.72 R123.1 15.75,90.89 v15.75,90.93
  Bottom 0.203: v8.26,87.76 7.48,88.53 7.48,90.93 | 7.48,90.93 USB101.SHIELD_TH1 | v15.75,90.93 7.48,90.93
XDSET_TCK_SWDCLK  (via drill 0.3)
  Top 0.203: IC106.P$35 25.62,68.11 26.42,67.31 26.42,64.26 v26.92,63.75 | v32,59.69 36.07,59.69 39.12,56.64 42.93,56.64 44.45,58.17 J102.4
  Bottom 0.203: v32,59.69 29.46,57.15 J101.16 29.21,60.2 26.92,62.48 v26.92,63.75
XDSET_TDI  (via drill 0.3)
  Top 0.203: IC106.P$38 27.78,69.31 v27.81,69.34 | v32.13,66.29 32.13,65.91 33.27,64.77 34.04,64.77 v35.81,62.99 | v35.81,61.47 39.88,57.4 41.4,57.4 41.91,57.91 J102.8
  Bottom 0.203: v27.81,69.34 30.61,69.34 31.75,68.2 31.75,66.67 v32.13,66.29 | J101.20 35.81,58.67 v35.81,61.47 v35.81,62.99
XDSET_TDO_SWO  (via drill 0.3)
  Top 0.203: IC106.P$37 26.47,68.91 27.43,67.95 27.43,65.66 28.32,64.77 28.32,62.61 v28.19,62.48 | v34.8,60.45 36.07,60.45 39.5,57.02 42.29,57.02 43.18,57.91 J102.6
  Bottom 0.203: J101.18 31.75,57.4 v34.8,60.45 30.23,60.45 v28.19,62.48
XDSET_TMS_SWDIO  (via drill 0.3)
  Top 0.203: IC106.P$36 26.1,68.51 26.92,67.69 26.92,65.41 27.81,64.52 27.81,63.12 27.18,62.48 v27.18,61.21 | J101.14 28.19,58.67 36.07,58.67 38.48,56.26 43.81,56.26 45.72,58.17 J102.2
  Bottom 0.203: v27.18,61.21 27.18,57.66 J101.14
XDSET_TXD  (via drill 0.3)
  Top 0.203: IC106.P$34 25.38,67.71 25.91,67.18 25.91,62.99 v25.65,62.74 | J101.8 23.11,61.21 v23.11,61.72
  Bottom 0.203: v23.11,61.72 24.13,62.74 v25.65,62.74
XDSET_VBAT  (via drill 0.3)
  Top 0.203: R104.2 C103.1 29.59,77.34 v29.46,77.47 | IC106.P$68 21.41,78.28 v21.97,77.72
  Bottom 0.203: v21.97,77.72 22.23,77.47 v29.46,77.47
XDSET_VBUS  (via drill 0.3, 0.51)
  Top 0.203: IC102.6 10.54,87.5 9.65,88.39 v9.65,88.65 9.75,88.74 | R132.1 8.8,60.54 v10.16,59.18
  Top 0.305: 53.86,83.44 C117.1 | T101.2 52.83,80.26 | IC101.5 22.23,87.58 | IC101.8 22.23,85.62
  Top 0.406: 22.23,85.62 22.23,87.58 21.31,87.58 C141.1 20.27,88.59 | USB101.VBUS 10.13,89.12 v9.65,88.65 6.86,88.65 6.1,87.88 6.1,87.25 C140.+ 4.8,83.9 R140.1 5.9,81.98 v6.35,81.53 | 20.27,88.59 20.22,88.65 v18.29,88.65 | R120.1 53.85,86.1 53.85,86.87 51.82,88.9 43.43,88.9 41.4,90.93 22.61,90.93 20.27,88.59
  Top 0.508: 52.83,80.26 52.35,80.54 51.84,80.92 v51.84,81.1 | C117.1 54.05,83.52 54.53,83.03 v54.53,82.32 54.58,82.27
  Top 0.61: R120.1 53.83,84.93 | C118.1 53.86,83.84
  Top 0.635: 53.83,84.93 C118.1 | 53.86,83.84 C117.1
  Bottom 0.203: v10.16,59.18 10.16,58.93 10.67,58.42
  Bottom 0.406: v6.35,81.53 6.35,78.23 2.54,74.42 2.54,58.17 3.81,56.9 9.14,56.9 10.67,58.42 12.7,58.42 J101.4 | v18.29,88.65 17.27,89.66 10.67,89.66 v9.65,88.65
  Bottom 0.508: v51.84,81.1 51.84,81.66 52.5,82.32 v54.53,82.32
XDSET_VCC  (via drill 0.3, 0.51)
  Top 0.203: 39.43,85.34 C124.1 | 39.43,86.84 C106.+ 39.37,86.86 | C104.1 12.76,63.49 C107.1 12.46,63.37 v11.43,63.37 | IC106.P$8 13.01,64.59 13.74,63.86 C104.1 | v7.11,74.93 7.11,74.11 C114.1 7.07,73.79 7.55,73.31 IC106.P$113 10.38,73.31 11.05,72.64 11.05,70.23 10.54,69.72 8.7,69.72 IC106.P$122 | v22.99,63.5 22.17,63.5 C112.1 21.78,63.57 21.01,64.33 IC106.P$28 21.01,66.75 20.83,66.93 20.45,66.93 20.21,66.69 IC106.P$26 | IC106.P$79 17.01,79.26 17.27,78.99 20.83,78.99 21.01,79.18 IC106.P$69 21.01,82.5 arc90 C121.1 21.68,82.58 v21.75,82.64 | IC106.P$90 12.61,80.11 10.61,78.11 IC106.P$101 6.87,78.11 C123.1 6.48,76.96 v6.6,76.84 | IC106.P$8 IC106.P$7 | IC106.P$16 16.21,67.48 15.88,67.82 13.34,67.82 13.01,67.49 IC106.P$8 | v29.34,72.14 29.31,72.11 C130.2 27.98,72.26 C113.1 | C113.1 26.93,72.26 | IC106.P$39 22.36,69.71 21.97,70.1 21.97,72.9 | 21.97,72.9 21.97,74.04 22.44,74.51 IC106.P$51 | IC106.P$51 IC106.P$52 | IC106.P$47 24.12,72.9 21.97,72.9 | R103.1 R104.1 v30.48,74.17 | C104.1 14.36,63.49 14.61,63.25 14.61,62.87 14.83,62.64 R105.2 | R125.2 3.61,82.51 R129.2 3.61,81.79 v2.92,81.79 | R116.1 39.66,76.9 R117.1 38.06,76.71 v37.85,76.71 37.72,76.58 R114.1 | IC106.P$51 25.42,74.51 26.16,73.77 26.16,72.52 26.42,72.26 27.17,72.26 C113.1 | R135.1 7.26,63.63 7.75,63.63 v8.26,64.14 | 28.45,82.56 v28.45,85.59 v28.45,85.6
  Top 0.305: MSP101.16 MSP101.15 39.43,85.34
  Top 0.406: IC101.1 27.27,85.62 | 54.38,69.97 C126.1 54.48,71.71 IC103.5
  Top 0.508: 54.38,69.97 v53.27,69.97
  Top 0.61: 39.43,85.34 39.43,86.84 | 39.37,86.86 v39.37,87.88
  Top 1.016: 28.58,83.07 28.58,82.56 28.96,82.56 28.96,85.86 27.27,85.86 27.27,85.62 27.27,84.36 C105.1 | 28.58,83.07 28.58,85.23 27.94,85.23 27.94,84.09 27.31,84.09 27.31,83.32 | 27.82,83.32 27.31,83.32 | 27.31,83.32 27.31,82.56 28.45,82.56 28.45,83.07 28.58,83.07
  other vias: 28.45,84.58 28.45,83.57 28.45,82.55
  pour Mid-Top (isolate 0.254): 0,95.25 58.42,95.25 58.42,56.64 0,56.64
XDSET_VCCOUT
  Top 0.203: 42.82,74.8 43.91,75.91 | 43.91,75.91 43.94,75.94 43.94,75.95 44.07,75.95 44.96,76.84 46.23,76.84 46.86,77.47 46.86,77.5 | 47.37,75.44 47.37,75.56 47.39,75.55 C120.1 | R112.1 43.91,75.9 43.91,75.91
  Top 0.305: R126.1 47.08,80.62 R128.1 47.08,79.11 46.79,78.82 46.79,77.71 R127.1 | 46.86,77.5 46.9,77.5 R127.1 | C120.1 47.53,75.99 46.96,76.56 46.96,77.54 R127.1
  Top 0.406: C119.1 52.57,75.94
  Top 0.508: 48.74,75.7 48.74,75.71 C127.1 48.77,75.61 48.76,75.61 | 52.57,75.94 IC103.3
  Top 0.635: 48.76,75.61 49.33,76.05 52.57,76.05 C119.1 52.59,76.02 52.6,76.02 | 48.74,75.7 47.75,75.69 47.75,75.62 C120.1 | L101.2 52.58,77.95 52.58,76.3 52.55,76.3 52.55,76.2 52.68,76.2 52.68,76.05 52.6,76.05 52.6,76.02 | 52.6,76 52.6,76.02
XDSET_VCCTARGET  (via drill 0.51)
  Top 0.203: R134.1 46.35,71.67 46.35,70.55
  Top 0.254: JP102.1 46.48,64.01 v41.15,64.01
  Top 0.508: IC103.4 50.69,71.73 50.67,71.7 C128.+ | 50.55,71.63 49.23,71.63 C129.1
  Top 0.61: C129.1 49.15,71.02 48.67,70.55 46.35,70.55 45.97,70.55 41.15,65.72 v41.15,64.01 v40.39,63.25
  Top 0.635: C128.+ 50.57,71.5 50.55,71.63
  Mid-Top 0.61: J101.6 18.03,58.67 35.81,58.67 v41.15,64.01
(copper drawn outside any net)
  shapes: Top area x2

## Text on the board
bPlace: J1 | J3 | J4 | J2
tDocu: TP101 | MSP432 Reset | Rev 2.1 | TP107 | XDS110 Out | MSP-EXP432P401R | XDS110-ET Rev 1.1 | Enable | XDS110 | Power | Out | RXD<< | TXD>> | RST | TMS | TCK | TDO | TDI | P1.1 | P1.4 | MSP432 In | P2.7 | P6.0 | P2.6 | P2.5 | P3.2 | P2.4 | P6.1 | P3.0 | P3.3 | P5.6 | P4.0 | P5.7 | P4.1 | P6.6 | P4.2 | !RST | P4.3 | P6.7 | P4.4 | P1.6 | P1.5 | P2.3 | P4.5 | P1.7 | P4.6 | P4.7 | P5.1 | P5.0 | P6.5 | P3.5 | P5.4 | P5.2 | P6.4 | P3.7 | P5.5 | P3.6 | Red P1.0 | Red P2.0 | Green P2.1 | Blue P2.2 | LED2 | LED1 | 8.5 | 9.0 | 8.4 | 8.2 | 9.2 | 6.2 | 7.3 | 7.1 | 9.4 | 9.6 | 8.0 | 7.4 | 7.6 | 10.0 | 10.2 | 10.4 | 8.6 | 8.7 | 9.1 | 8.3 | 5.3 | 9.3 | 6.3 | 7.2 | 7.0 | 9.5 | 9.7 | 7.5 | 7.7 | 10.1 | 10.3 | 10.5
bDocu: P2.7 | P2.5 | P6.0 | P2.6 | P6.1 | P3.0 | P3.2 | P2.4 | P4.0 | P5.7 | P3.3 | P5.6 | P4.2 | !RST | P4.1 | P6.6 | P4.4 | P1.6 | P4.3 | P6.7 | P4.5 | P1.7 | P1.5 | P2.3 | P4.7 | P4.6 | P5.0 | P5.1 | P5.4 | P5.2 | P6.5 | P3.5 | P5.5 | P3.6 | P6.4 | P3.7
